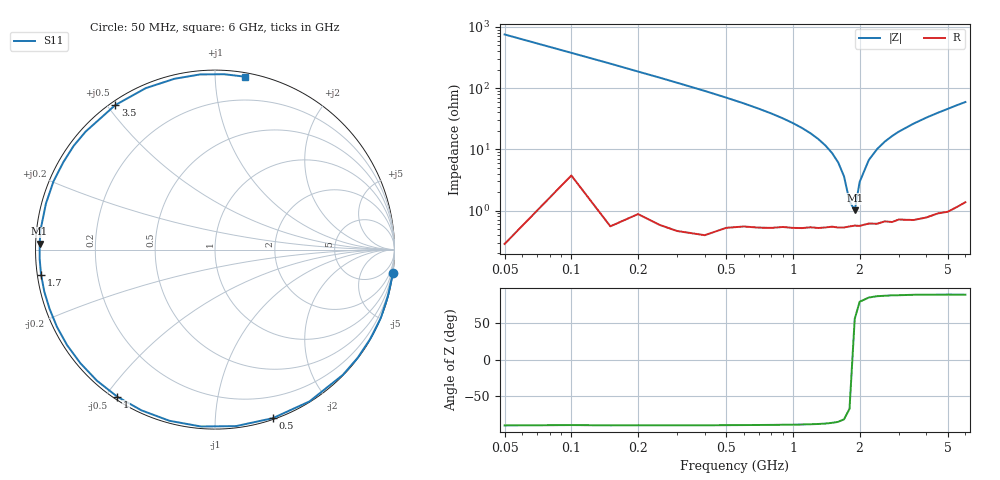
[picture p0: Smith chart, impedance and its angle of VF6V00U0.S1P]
! Infineon Technologies  Discrete & RF Semiconductors
! BBY 58-03
! Si Tuning Diode in SOD323
! VR = 6 V
! S-Parameters:  June  1999
# GHz  S  MA  R  50
!  f  S11
! GHz  MAG  ANG
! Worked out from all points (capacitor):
!   34 points, 50 MHz to 6 GHz, reference 50 ohm
!   read as one part to ground: C = 4.21 pF near 50 MHz
!   lowest |Z| = 1 ohm at 1.9 GHz (marker M1)
!   series resonance near 1.861 GHz, so ESL is about 1.7 nH
!   S11 on the Smith chart (normalised r, x): 50 MHz: 0, -15; 500 MHz: 0.01, -1.40; 1 GHz: 0.01, -0.54; 1.7 GHz: 0.01, -0.07; 3.5 GHz: 0.01, +0.52; 6 GHz: 0.03, +1.19
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0.05  1 -7.6
0.15  0.9992 -22.5
0.25  0.9976 -37.2
0.3  0.9974 -44.4
0.4  0.9963 -58.1
0.5  0.993 -71.1
0.6  0.9904 -83.2
0.7  0.9887 -94.5
0.8  0.987 -104.9
0.9  0.9849 -114.6
1  0.984 -123.6
1.1  0.9829 -132.0
1.2  0.9814 -139.8
1.3  0.9811 -147.1
1.4  0.9801 -153.9
1.6  0.9795 -166.1
1.7  0.9792 -171.8
1.9  0.9776 178.1
2.2  0.9762 164.8
2.4  0.9769 157.1
2.6  0.9754 150.0
3  0.9755 137.6
3.5  0.9783 124.6
4  0.9788 113.2
4.5  0.9782 103.4
5  0.9795 94.9
5.5  0.9785 87.0
6  0.9775 80.3
